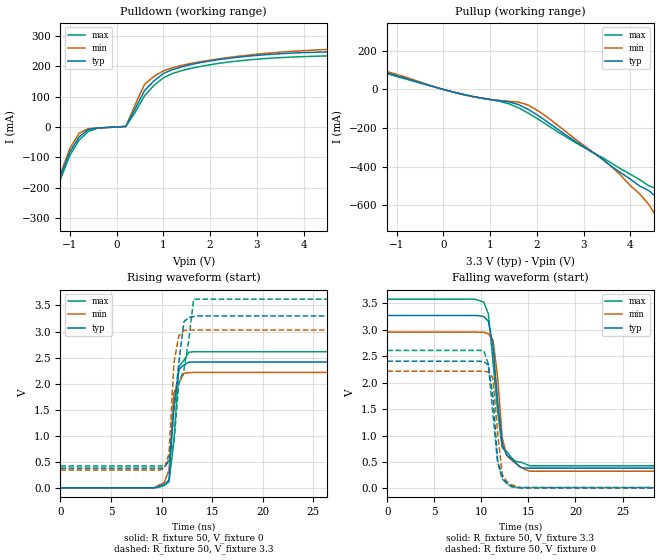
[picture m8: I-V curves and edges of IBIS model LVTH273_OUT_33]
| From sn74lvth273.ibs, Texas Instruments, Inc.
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|   Model LVTH273_OUT_33
[Model]   LVTH273_OUT_33
Model_type  Output
Polarity   Non-Inverting
Vmeas = 1.5V
Cref = 50pf
Rref = 500
Vref = 0V
| variable   typ   min   max
C_comp   7p   NA   NA
[Temperature Range]   40   -25   100
| Ambient temperature   25   -40   85
[Voltage range]   3.3   3.0   3.6
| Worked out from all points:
|   slope of the pulldown table from 0 to 0.495 V, typ, clamps not added: 5.54 ohm
|   slope of the pullup table from 0 to 0.495 V, typ, clamps not added: 16.8 ohm
|   rising waveform, R_fixture 50, V_fixture 0: 20-80 % time 625ps typ, 436ps min, 646ps max; typ from 0.012 V to 2.42 V
|   falling waveform, R_fixture 50, V_fixture 3.3: 20-80 % time 906ps typ, 867ps min, 1.08ns max; typ from 3.27 V to 0.384 V
|   rising waveform, R_fixture 50, V_fixture 3.3: 20-80 % time 946ps typ, 513ps min, 1.47ns max; typ from 0.386 V to 3.3 V
|   falling waveform, R_fixture 50, V_fixture 0: 20-80 % time 721ps typ, 716ps min, 828ps max; typ from 2.41 V to 0.01 V
[Pulldown]
|   Voltage   I(typ)   I(min)   I(max)
-5V       -3.148A    -3.573A    -2.751A
-1.6V     -383.5mA   -394.9mA   -425.8mA
-1.4V     -261mA     -265.3mA   -286.8mA
-1.2V     -160.6mA   -155.2mA   -172.7mA
-800mV    -32.49mA   -20.37mA   -43.22mA
-400mV    -3.29mA    -3.605mA   -3.725mA
200mV     1.743mA    1.631mA    1.96mA
600mV     120.2mA    140.4mA    103mA
1V        176.2mA    185mA      161.8mA
1.4V      198.5mA    203.2mA    185.9mA
3.4V      240.6mA    245.4mA    227.7mA
10V       282.7mA    336.3mA    261.8mA
[Pullup]
|   Voltage   I(typ)   I(min)   I(max)
-5V       303.2mA    316.2mA    292.5mA
-2.4V     165.4mA    178mA      159.3mA
400mV     -24.45mA   -25.42mA   -24.06mA
1.4V      -64.76mA   -61.06mA   -74.28mA
1.8V      -101.2mA   -79.43mA   -120.5mA
3.6V      -399.6mA   -401.5mA   -382.9mA
4.4V      -525.9mA   -598.6mA   -500.5mA
4.6V      -567.1mA   -678.3mA   -518.6mA
4.8V      -629mA     -762.8mA   -552.4mA
5V        -703.4mA   -847.3mA   -603.3mA
5.4V      -855.4mA   -1.016A    -732.3mA
10V       -2.603A    -2.96A     -2.298A
[Ramp]
| variable   typ   min   max
dV/dt_r  1.476E+00/5.380E-10  1.356E+00/5.230E-10  1.614E+00/5.570E-10
dV/dt_f  1.728E+00/7.220E-10  1.566E+00/6.160E-10  1.882E+00/8.200E-10
R_load = 50
[Rising Waveform]
R_fixture = 50
V_fixture = 0
V_fixture_min = 0
V_fixture_max = 0
C_fixture = 0pf
L_fixture = 0nH
|   Time   V(typ)   V(min)   V(max)
0s        11.64mV    11.94mV    10.38mV
9.277ns   11.64mV    11.94mV    10.38mV
9.766ns   41.76mV    65.18mV    21.73mV
10.25ns   71.66mV    108mV      55.58mV
10.74ns   158.2mV    344.5mV    122.8mV
11.23ns   1.583V     1.834V     917.5mV
11.72ns   2.276V     2.021V     2.33V
12.21ns   2.359V     2.2V       2.449V
12.7ns    2.415V     2.214V     2.604V
49.71ns   2.418V     2.219V     2.614V
[Falling Waveform]
R_fixture = 50
V_fixture = 3.3
V_fixture_min = 3
V_fixture_max = 3.6
C_fixture = 0pf
L_fixture = 0nH
|   Time   V(typ)   V(min)   V(max)
0s        3.272V     2.959V     3.582V
10.25ns   3.252V     2.956V     3.525V
10.74ns   3.166V     2.925V     3.303V
11.23ns   2.696V     2.808V     2.403V
11.72ns   1.674V     2.115V     1.478V
12.21ns   837.1mV    957.4mV    766.5mV
12.7ns    627.9mV    620.3mV    696.3mV
13.67ns   480.2mV    470.7mV    504.9mV
15.14ns   383.6mV    325.6mV    428.1mV
49.71ns   383.6mV    325.6mV    428.1mV
[Rising Waveform]
R_fixture = 50
V_fixture = 3.3
V_fixture_min = 3
V_fixture_max = 3.6
C_fixture = 0pf
L_fixture = 0nH
|   Time   V(typ)   V(min)   V(max)
0s        386.3mV    349.2mV    427.7mV
9.766ns   386.3mV    349.2mV    427.7mV
10.25ns   391.8mV    375.5mV    434.8mV
10.74ns   529.8mV    662.7mV    539.9mV
11.23ns   1.498V     2.403V     877.9mV
11.72ns   2.425V     2.924V     2.027V
12.21ns   3.186V     3.022V     2.259V
12.7ns    3.27V      3.03V      2.845V
13.18ns   3.289V     3.03V      3.621V
49.71ns   3.3V       3.03V      3.621V
[Falling Waveform]
R_fixture = 50
V_fixture = 0
V_fixture_min = 0
V_fixture_max = 0
C_fixture = 0pf
L_fixture = 0nH
|   Time   V(typ)   V(min)   V(max)
0s        2.407V     2.217V     2.611V
10.25ns   2.4V       2.213V     2.607V
10.74ns   2.336V     2.205V     2.351V
11.23ns   1.726V     2.086V     1.389V
11.72ns   534.5mV    1.062V     500mV
12.21ns   214.7mV    265.5mV    178.6mV
12.7ns    93.09mV    128.8mV    95.22mV
13.18ns   45.46mV    69.1mV     31.28mV
14.16ns   10.14mV    12.09mV    18.79mV
49.71ns   10.14mV    12.09mV    18.79mV
